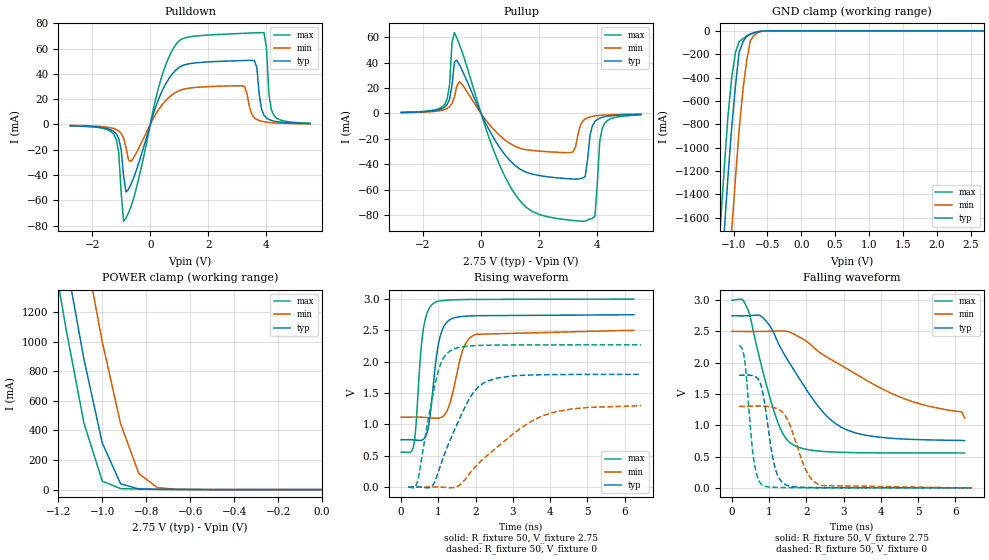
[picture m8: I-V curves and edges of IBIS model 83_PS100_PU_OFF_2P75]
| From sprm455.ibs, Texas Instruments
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|   Model Cell 83_PS100_PU_OFF_2P75
|IDG09_OUI83_PS100_PU_OFF_2P75
[Model]   83_PS100_PU_OFF_2P75
Model_type   I/O
Polarity   Non-Inverting
Enable   Active-Low
Vinl =  0.7V
Vinh =  1.7V
Cref =  15pF
Rref =  100.00M
Vref =  0V
Vmeas =  1.375
C_comp   4.835p   4.751p   5.207p
[Model Spec]
Vinl   0.7V   0.7V   0.7V
Vinh   1.7V   1.7V   1.7V
[Temperature Range]   25   125   -40
[Voltage Range]   2.75   2.5   3
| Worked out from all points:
|   slope of the pulldown table from 0 to 0.412 V, typ, clamps not added: 15.5 ohm
|   slope of the pullup table from 0 to 0.412 V, typ, clamps not added: 22.4 ohm
|   GND clamp passes 1 mA (typ) near -0.51 V on its own axis
|   POWER clamp passes 1 mA (typ) near -0.68 V on its own axis
|   rising waveform, R_fixture 50, V_fixture 2.75: 20-80 % time 246ps typ, 342ps min, 189ps max; typ from 0.754 V to 2.75 V
|   rising waveform, R_fixture 50, V_fixture 0: 20-80 % time 799ps typ, 1.58ns min, 433ps max; typ from 0 V to 1.8 V
|   falling waveform, R_fixture 50, V_fixture 2.75: 20-80 % time 1.32ns typ, 2.55ns min, 662ps max; typ from 2.75 V to 0.754 V
|   falling waveform, R_fixture 50, V_fixture 0: 20-80 % time 289ps typ, 476ps min, 204ps max; typ from 1.8 V to 0 V
| Nom Voltages:
|   VDD=1.1, VDDS=2.75, VSS=0, VSSS=0
| Min Voltages:
|   VDD=1, VDDS=2.5, VSS=0, VSSS=0
| Max Voltages:
|   VDD=1.2, VDDS=3, VSS=0, VSSS=0
[POWER_clamp]
|   voltage   I(typ)   I(min)   I(max)
-2.75V    16.79A     17.52A     16.39A
-1.194V   1.811A     2.617A     1.344A
-1.139V   1.338A     2.134A     883.7mA
-1.083V   881.6mA    1.66A      449.6mA
-1.056V   692.8mA    1.44A      318.6mA
-1.028V   503.9mA    1.22A      187.7mA
-1V       315.1mA    1.001A     56.76mA
-916.7mV  39.37mA    445.9mA    6.56mA
-833.3mV  4.345mA    107.2mA    3.75mA
-750mV    1.777mA    13.92mA    2.234mA
-666.7mV  898uA      2.213mA    1.085mA
0V        78.35pA    12.43nA    963.7fA
[Pulldown]
|   voltage   I(typ)   I(min)   I(max)
-2.75V    -951.5uA   -727.1uA   -1.064mA
-1.25V    -5.613mA   -3.252mA   -7.974mA
-1.083V   -11.23mA   -5.133mA   -21.99mA
-916.7mV  -40.86mA   -10.78mA   -76.55mA
-666.7mV  -47.43mA   -29.33mA   -65.21mA
333.3mV   22.59mA    13.28mA    33.12mA
1.083V    46.33mA    27.47mA    67.49mA
3.167V    50.55mA    30.63mA    72.03mA
3.583V    50.51mA    5.33mA     72.45mA
3.917V    7.298mA    2.134mA    72.52mA
4.25V     2.705mA    1.306mA    7.402mA
5.5V      771.4uA    522.6uA    1.048mA
[Pullup]
|   voltage   I(typ)   I(min)   I(max)
-2.75V    781.9uA    636.2uA    897.4uA
-1.25V    5.061mA    3.14mA     7.247mA
-1.083V   11.26mA    5.325mA    22.87mA
-916.7mV  40.27mA    13.02mA    63.52mA
-750mV    38.45mA    24.96mA    54.5mA
1.167V    -40.69mA   -25.69mA   -63.3mA
3.167V    -51.47mA   -30.16mA   -84mA
3.5V      -50.78mA   -6.037mA   -84.66mA
3.917V    -6.314mA   -1.951mA   -80.81mA
4.083V    -3.692mA   -1.517mA   -21.92mA
4.25V     -2.581mA   -1.238mA   -7.85mA
5.5V      -773uA     -514.5uA   -1.206mA
[GND_clamp]
|   voltage   I(typ)   I(min)   I(max)
-2.75V    -17.23A    -18.11A    -16.74A
-1.194V   -2.218A    -3.158A    -1.668A
-1.139V   -1.732A    -2.663A    -1.193A
-1.083V   -1.257A    -2.175A    -737.7mA
-1.028V   -833.1mA   -1.71A     -401.9mA
-972.2mV  -474.8mA   -1.266A    -186.1mA
-916.7mV  -182.2mA   -842.6mA   -90.42mA
-861.1mV  -95.88mA   -507.3mA   -67.05mA
-805.6mV  -43.79mA   -253.3mA   -46.5mA
-750mV    -25.96mA   -80.64mA   -28.77mA
-472.2mV  -313.8uA   -1.032mA   -106.8uA
2.694V    74.94pA    440.3nA    648.4fA
[Ramp]
| variable   typ   min   max
dV/dt_f  1.2052463/1.3253086n  0.8363043/2.5501857n  1.4753653/0.66464611n
dV/dt_r  1.0874342/0.80180066n 0.78850335/1.5831186n  1.3704481/0.43510226n
R_load = 50
[Rising Waveform]
R_fixture = 50
V_fixture = 2.75
V_fixture_min = 2.5
V_fixture_max = 3
|   time   V(typ)   V(min)   V(max)
0s        753.7mV    1.115V     557.4mV
337.6ps   751.7mV    1.116V     664.5mV
594.5ps   760mV      1.113V     2.511V
741.8ps   992.6mV    1.107V     2.84V
890.2ps   1.784V     1.099V     2.942V
1.02ns    2.335V     1.101V     2.969V
1.182ns   2.598V     1.167V     2.98V
1.669ns   2.725V     2.209V     2.993V
2.008ns   2.735V     2.438V     2.996V
6.25ns    2.75V      2.5V       3V
[Rising Waveform]
R_fixture = 50
V_fixture = 0
V_fixture_min = 0
V_fixture_max = 0
|   time   V(typ)   V(min)   V(max)
190.4ps   0V         0V         0V
440ps     0V         0V         86.83mV
843.2ps   23.11mV    0V         1.441V
1.044ns   321mV      0V         1.936V
1.332ns   770.4mV    -11.91mV   2.178V
1.899ns   1.472V     259.2mV    2.255V
2.348ns   1.698V     521.4mV    2.264V
3.401ns   1.787V     1.014V     2.269V
4.046ns   1.794V     1.185V     2.269V
6.44ns    1.799V     1.302V     2.27V
[Falling Waveform]
R_fixture = 50
V_fixture = 2.75
V_fixture_min = 2.5
V_fixture_max = 3
|   time   V(typ)   V(min)   V(max)
0s        2.75V      2.5V       3V
270.5ps   2.749V     2.5V       3.012V
433.6ps   2.751V     2.499V     2.841V
774.4ps   2.747V     2.5V       1.991V
1.127ns   2.47V      2.504V     1.228V
1.382ns   2.158V     2.508V     851.5mV
1.634ns   1.912V     2.467V     690.7mV
2.436ns   1.218V     2.131V     582.9mV
3.071ns   929.2mV    1.91V      565.7mV
6.25ns    753.7mV    1.115V     557.4mV
[Falling Waveform]
R_fixture = 50
V_fixture = 0
V_fixture_min = 0
V_fixture_max = 0
|   time   V(typ)   V(min)   V(max)
190.4ps   1.799V     1.302V     2.27V
340.6ps   1.803V     1.302V     2.036V
528.4ps   1.797V     1.306V     736.4mV
603.6ps   1.783V     1.307V     383.5mV
823.3ps   1.531V     1.308V     42.54mV
1.147ns   345.8mV    1.278V     8.287mV
1.444ns   49.62mV    1.143V     4.749mV
1.984ns   7.375mV    287mV      2.074mV
2.317ns   4.52mV     57.84mV    0V
6.44ns    0V         0V         0V
